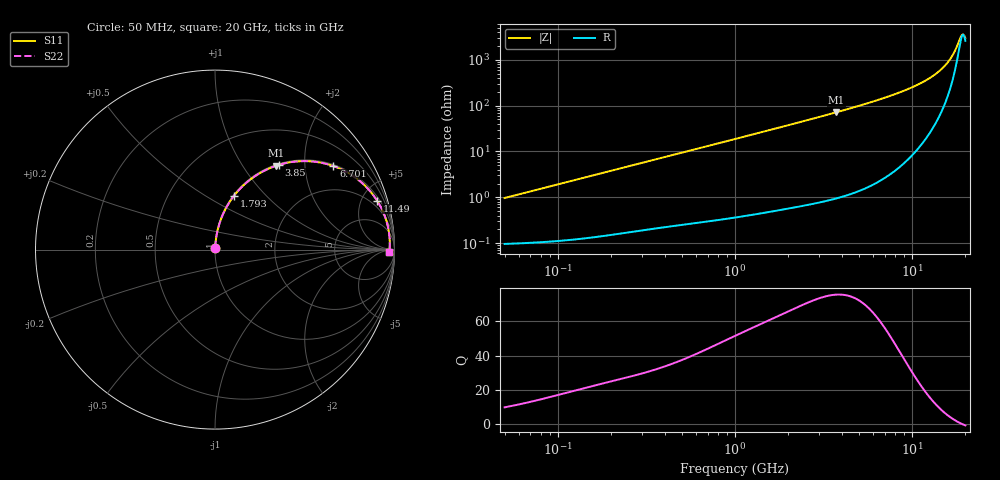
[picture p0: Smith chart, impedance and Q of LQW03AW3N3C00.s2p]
!Murata Part Number: LQW03AW3N3C00
!These Parameters are Measured in Series Mode Connection
!  o--[Z]--o
!Port1  Port2
!  o-------o
!Freq. Start=50[MHz] Stop=20[GHz], 401[Steps]
# Hz S RI R 50
!Freq.(Hz) S11(Real) S11(Imag) S21(Real) S21(Imag) S12(Real) S12(Imag) S22(Real) S22(Imag)
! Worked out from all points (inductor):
!   401 points, 50 MHz to 20 GHz, reference 50 ohm
!   read as one part in series: L = 3.05 nH near 51.52 MHz
!   highest Q = 75.6 at 3.736 GHz (marker M1), where L = 3.05 nH
!   self-resonance near 19.42 GHz
!   S11 on the Smith chart (normalised r, x): 50 MHz: 1.00, +0.02; 1.793 GHz: 1.01, +0.67; 3.85 GHz: 1.02, +1.48; 6.701 GHz: 1.05, +2.80; 11.49 GHz: 1.31, +6.50; 20 GHz: 53, -29
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5e7  0.00105 0.00958  0.9989 -0.00958  0.9989 -0.00958  0.00105 0.00958
1.364002e8  0.00192 0.0259  0.9981 -0.0259  0.9981 -0.0259  0.00192 0.0259
3.721004e8  0.00699 0.0694  0.993 -0.0694  0.993 -0.0694  0.00699 0.0694
6.285508e8  0.0163 0.1153  0.9837 -0.1153  0.9837 -0.1153  0.0163 0.1153
1e9  0.0369 0.1789  0.9631 -0.1789  0.9631 -0.1789  0.0369 0.1789
1.793498e9  0.1046 0.2982  0.8954 -0.2982  0.8954 -0.2982  0.1046 0.2982
2.728004e9  0.212 0.4019  0.788 -0.4019  0.788 -0.4019  0.212 0.4019
3.736399e9  0.3404 0.4673  0.6596 -0.4673  0.6596 -0.4673  0.3404 0.4673
3.850025e9  0.3548 0.4719  0.6452 -0.4719  0.6452 -0.4719  0.3548 0.4719
5.117541e9  0.5062 0.493  0.4938 -0.493  0.4938 -0.493  0.5062 0.493
6.701223e9  0.6598 0.4654  0.3402 -0.4654  0.3402 -0.4654  0.6598 0.4654
7.442007e9  0.7169 0.441  0.2831 -0.441  0.2831 -0.441  0.7169 0.441
9.457416e9  0.8319 0.3597  0.1681 -0.3597  0.1681 -0.3597  0.8319 0.3597
1.149051e10  0.9031 0.2731  0.0969 -0.2731  0.0969 -0.2731  0.9031 0.2731
1.354865e10  0.9446 0.1907  0.0554 -0.1907  0.0554 -0.1907  0.9446 0.1907
1.527346e10  0.9635 0.1277  0.0365 -0.1277  0.0365 -0.1277  0.9635 0.1277
1.621653e10  0.9694 0.0958  0.0306 -0.0958  0.0306 -0.0958  0.9694 0.0958
1.696185e10  0.9722 0.0719  0.0278 -0.0719  0.0278 -0.0719  0.9722 0.0719
1.88369e10  0.9736 0.0161  0.0264 -0.0161  0.0264 -0.0161  0.9736 0.0161
1.912117e10  0.9732 0.00814  0.0268 -0.00814  0.0268 -0.00814  0.9732 0.00814
1.940974e10  0.9727 0.000249  0.0273 -0.000249  0.0273 -0.000249  0.9727 0.000249
2e10  0.9711 -0.0155  0.0289 0.0155  0.0289 0.0155  0.9711 -0.0155
